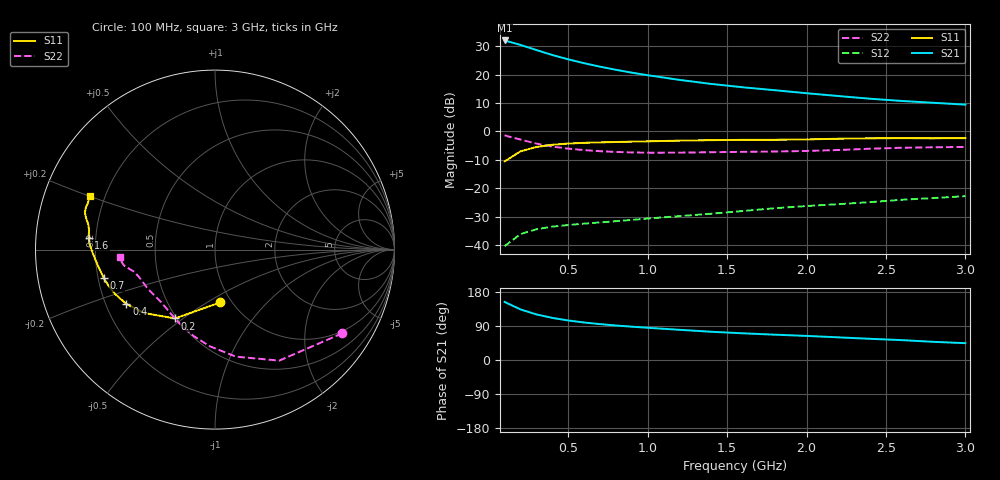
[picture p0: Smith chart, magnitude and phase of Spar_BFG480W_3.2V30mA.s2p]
! Filename: 3_230BFG480.001
! Title: BFG480W
! Bias: Vce=3.2V; Ic=30mA
! Company: NXP Semiconductors NL
! User: Quality&Reliability T&D
! Measure time: 10 Nov 1999 / 11:56:35
#  MHz  S  MA  R 50
! Freq  S11  S21  S12  S22  :
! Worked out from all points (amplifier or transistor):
!   20 points, 100 MHz to 3 GHz, reference 50 ohm
!   highest |S21| = 32.0 dB at 100 MHz (marker M1)
!   |S21| within 3 dB of that: start of sweep to 279.3 MHz
!   unconditionally stable (mu >= 1): 1.172 GHz to end of sweep
!   at 400 MHz: K = 0.50, MSG = 30.2 dB, |S12| = -33.6 dB
!   at 1.2 GHz: K = 1.01, MAG = 23.4 dB, |S12| = -29.9 dB
!   at 3 GHz: K = 1.09, MAG = 14.3 dB, |S12| = -22.8 dB
!   S11 on the Smith chart (normalised r, x): 100 MHz: 0.89, -0.57; 200 MHz: 0.49, -0.47; 400 MHz: 0.29, -0.26; 700 MHz: 0.22, -0.12; 1.6 GHz: 0.17, +0.05; 3 GHz: 0.14, +0.20
100  0.2954 -84.0  39.78 153.2  0.009507 67.0  0.8488 -33.4
200  0.4438 -120.2  33.21 133.5  0.01553 54.7  0.7147 -59.9
300  0.5307 -138.3  26.97 120.3  0.01885 48.9  0.6076 -79.0
400  0.5792 -148.5  22.05 111.1  0.02097 46.3  0.5392 -93.1
500  0.6089 -155.9  18.52 104.3  0.0224 45.8  0.4955 -104.0
600  0.6269 -161.3  15.82 99.0  0.0237 46.1  0.4669 -112.3
700  0.639 -165.5  13.76 94.7  0.02489 47.6  0.4471 -119.0
800  0.6485 -169.0  12.12 91.0  0.02619 49.4  0.4335 -124.7
900  0.6577 -172.0  10.78 87.9  0.02754 51.5  0.4249 -129.5
1000  0.667 -174.7  9.719 85.1  0.02912 53.4  0.4203 -134.0
1200  0.6849 -179.2  8.046 79.7  0.03212 56.9  0.4215 -141.4
1400  0.6993 177.5  6.83 74.5  0.03542 59.8  0.4289 -147.1
1600  0.7072 174.6  5.957 70.4  0.03957 62.7  0.4349 -151.4
1800  0.7094 171.5  5.295 66.8  0.04428 65.1  0.441 -155.7
2000  0.7202 168.7  4.683 63.6  0.04835 67.0  0.4511 -160.6
2200  0.7403 166.1  4.181 59.8  0.05221 68.3  0.469 -164.9
2400  0.7543 164.0  3.748 55.9  0.05667 68.9  0.4938 -167.9
2600  0.7564 162.1  3.424 52.5  0.06237 69.2  0.5137 -169.9
2800  0.7545 159.7  3.178 47.9  0.06693 68.6  0.5235 -172.1
3000  0.7598 156.9  2.949 44.4  0.07212 68.6  0.5315 -175.3
